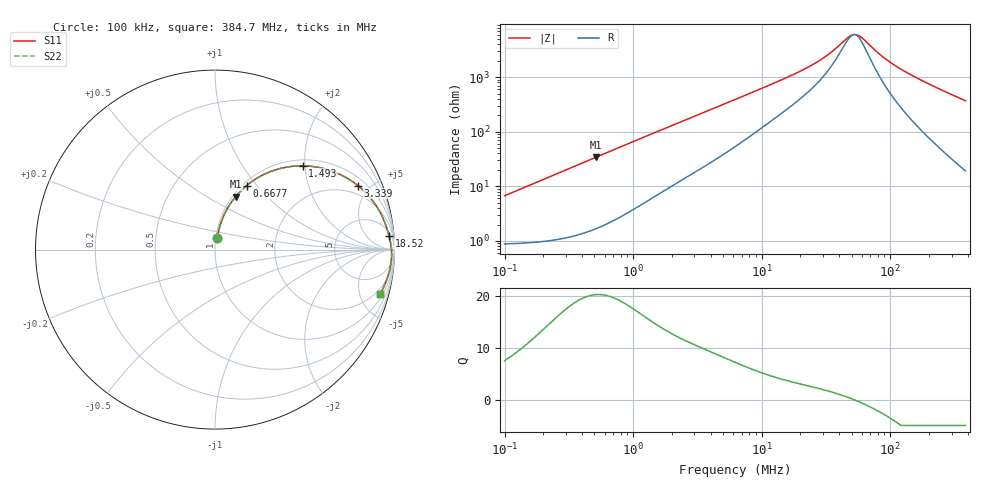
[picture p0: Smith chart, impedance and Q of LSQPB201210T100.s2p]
! LSQPB201210T100  S-PARAMETER MODEL  ( General Type )
! Model Generated by TAIYO YUDEN Corporation (http://www.ty-top.com)
! Version 2.0
! TAIYO YUDEN Control No. 100810NF18SB-HKC
! Copyright(c) 2007 TAIYO YUDEN CO.,LTD. All Rights Reserved.
! Product Description (link to TY-COMPAS)
! https://ds.yuden.co.jp/TYCOMPAS/or/detail?pn=LSQPB201210T100M&u=M
! Products Name : Inductors
! Characteristics :
!  Inductance : 10 uH , SRF(min) : 30 MHz , DC Resistance(max) : 1.105 Ohm
!  Rated Current : Saturation :270 mA , Temp Rise : 330 mA (40 degC)
!  Case Size : 2.0 x 1.25 / 0.079 x 0.049 [mm/inch] , Thickness : 1.0 / 0.04 [mm/inch]
!  (Conditions: Temperature = 25 degC , DC Bias Current/Voltage = 0A / 0V)
! External Node Assignments :
!  1  o---GGG---o  2
! GND o---------o GND
! Frequency Range : 0.1MHz  -  384.651195MHz  [ 402 STEP ]
# MHz S RI R 50
! Freq[MHz].  S11 Real  S11 Imag  S21 Real  S21 Imag  S12 Real  S12 Imag  S22 Real  S22 Imag
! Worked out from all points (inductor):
!   401 points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, 100 kHz to 384.7 MHz, reference 50 ohm
!   read as one part in series: L = 10.6 uH near 104.2 kHz
!   highest Q = 20.3 at 510.6 kHz (marker M1), where L = 10.6 uH
!   self-resonance near 52.18 MHz
!   S11 on the Smith chart (normalised r, x): 100 kHz: 1.02, +0.13; 667.7 kHz: 1.04, +0.88; 1.493 MHz: 1.13, +1.95; 3.339 MHz: 1.42, +4.22; 18.52 MHz: 8, +22; 384.7 MHz: 1.38, -7.38
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0.1  0.013 0.0651  0.987 -0.0651  0.987 -0.0651  0.013 0.0651
0.205918  0.0277 0.132  0.9723 -0.132  0.9723 -0.132  0.0277 0.132
0.398565  0.0764 0.2414  0.9236 -0.2414  0.9236 -0.2414  0.0764 0.2414
0.510565  0.1147 0.2951  0.8853 -0.2951  0.8853 -0.2951  0.1147 0.2951
0.667675  0.1759 0.3565  0.8241 -0.3565  0.8241 -0.3565  0.1759 0.3565
1.051342  0.3331 0.4432  0.6669 -0.4432  0.6669 -0.4432  0.3331 0.4432
1.493171  0.4881 0.4669  0.5119 -0.4669  0.5119 -0.4669  0.4881 0.4669
1.588538  0.5161 0.4658  0.4839 -0.4658  0.4839 -0.4658  0.5161 0.4658
2.351192  0.6816 0.4256  0.3184 -0.4256  0.3184 -0.4256  0.6816 0.4256
3.339285  0.7956 0.3569  0.2044 -0.3569  0.2044 -0.3569  0.7956 0.3569
6.331348  0.9126 0.2209  0.0874 -0.2209  0.0874 -0.2209  0.9126 0.2209
10.60628  0.951 0.1377  0.049 -0.1377  0.049 -0.1377  0.951 0.1377
18.51633  0.9694 0.0768  0.0306 -0.0768  0.0306 -0.0768  0.9694 0.0768
24.71908  0.9752 0.053  0.0248 -0.053  0.0248 -0.053  0.9752 0.053
33.68777  0.9798 0.0303  0.0202 -0.0303  0.0202 -0.0303  0.9798 0.0303
47.84512  0.9831 0.00602  0.0169 -0.00602  0.0169 -0.00602  0.9831 0.00602
53.0458  0.9837 -0.00116  0.0163 0.00116  0.0163 0.00116  0.9837 -0.00116
60.03811  0.9842 -0.00992  0.0158 0.00992  0.0158 0.00992  0.9842 -0.00992
80.15015  0.9843 -0.0316  0.0157 0.0316  0.0157 0.0316  0.9843 -0.0316
98.5215  0.9834 -0.0487  0.0166 0.0487  0.0166 0.0487  0.9834 -0.0487
171.9979  0.9746 -0.1071  0.0254 0.1071  0.0254 0.1071  0.9746 -0.1071
384.6512  0.9208 -0.2453  0.0792 0.2453  0.0792 0.2453  0.9208 -0.2453
